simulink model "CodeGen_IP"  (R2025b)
settings: Solver=VariableStepAuto  StartTime=0.0  StopTime=10  RelTol=1e-3  EnableMultiTasking=on
undefined symbols (not defined in the file or in its folder): gray
libraries: hlsBasic x5, Sobeledge_lib x2, visionsinks x2, dspvision x1

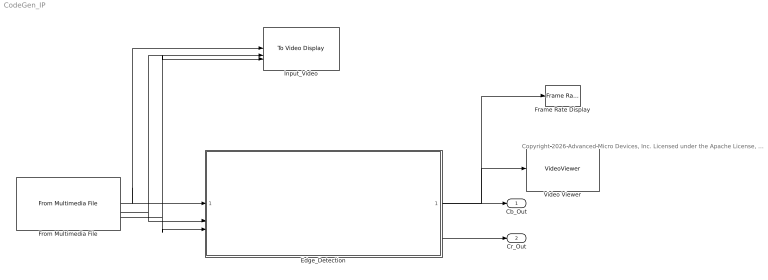
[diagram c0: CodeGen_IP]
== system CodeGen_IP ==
  note: Copyright 2026 Advanced Micro Devices, Inc. Licensed under the Apache License, Version 2.0 (the "License"); you may not use this file except in compliance with the License. You may obtain a copy of the License at http://www.apache.org/licenses/LICENSE-2.0 Unless required by applicable law or agreed to in writing, software distributed under the License is distributed on an "AS IS" BASIS, WITHOUT WARRANTIES OR CONDITIONS OF ANY KIND, either express or implied. See the License for the specific language governing permissions and limitations under the License.
  Edge_Detection : Subsystem
  Frame Rate Display : visionsinks/Frame Rate Display  UpdateRate=10
  From Multimedia File : dspvision/From Multimedia File  inputFilename=visiontraffic.avi  readRange=[1 Inf]  loop=on  numPlays=inf  outputStreams=Video only  videoDataType=uint8  audioDataType=int16  inheritSampleTime=off  userDefinedSampleTime=1/30  noAudioOutput=off  isIntensityVideo=off  fourcc=YCbCr 4:2:2  colorVideoFormat=Separate color signals  outputEOF=off  dataOrg=Column-major  audioFrameSize=1024  computeAudioFrameSize=off  outSamplingMode=Sample based
  Input_Video : visionsinks/To Video Display  windowSizeMode=Normal  openAtMdlStart=on  fullScreen=off  videoWindowX=150  videoWindowY=269  saveWindowSize=off  videoWindowWidth=581  videoWindowHeight=403  inputColorFormat=YCbCr 4:2:2  inputType=Obsolete  imagePorts=One multidimensional signal  OutputDevice=On-screen video monitor  dataOrg=Column-major  isWindowOpen=off
  Video Viewer : VideoViewer  colormapValue=gray(256)  FigPos=[755.4 772 579.6 322.8]
  Cb_Out : Outport
  Cr_Out : Outport  Port=2
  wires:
  From Multimedia File/1 -> Input_Video/1, Edge_Detection/1(Y)
  Edge_Detection/1(Y_Out) -> Video Viewer/1, Frame Rate Display/1
  From Multimedia File/2 -> Input_Video/2, Edge_Detection/2(Cb)
  From Multimedia File/3 -> Input_Video/3, Edge_Detection/3(Cr)
  Edge_Detection/3(Cr_Out) -> Cr_Out/1
  Edge_Detection/2(Cb_Out) -> Cb_Out/1

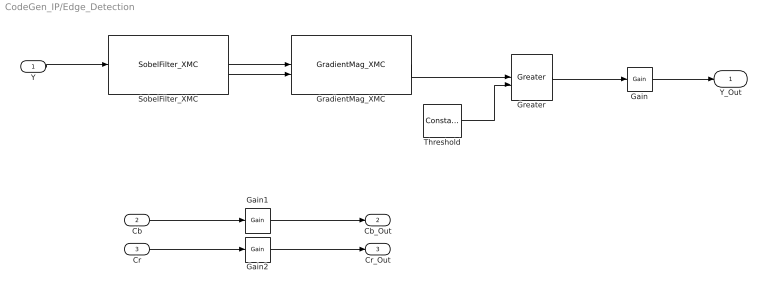
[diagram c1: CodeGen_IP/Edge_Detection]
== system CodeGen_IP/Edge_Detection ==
  Y : Inport
  Cb : Inport  Port=2
  Cr : Inport  Port=3
  Gain : hlsBasic/Gain  Gain=255  OutDataType=uint8  TypeExp=''  Signedness=Signed  WordLength=16  FractionalLength=10  RoundingMode=Truncation to minus infinity  OverflowMode=Wrap around  OutputTypeAsInput=off
  Gain1 : hlsBasic/Gain  Gain=1  OutDataType=uint8  TypeExp=''  Signedness=Signed  WordLength=16  FractionalLength=10  RoundingMode=Truncation to minus infinity  OverflowMode=Wrap around  OutputTypeAsInput=off
  Gain2 : hlsBasic/Gain  Gain=1  OutDataType=uint8  TypeExp=''  Signedness=Signed  WordLength=16  FractionalLength=10  RoundingMode=Truncation to minus infinity  OverflowMode=Wrap around  OutputTypeAsInput=off
  GradientMag_XMC : Sobeledge_lib/GradientMag_XMC  LibraryFunction=GradientMag_XMC  IncludeFiles={'GradientMag_Wrap.h'}  SourceFiles={}  IncludeDirectories={'./include'}  TemplateParams={'int ROWS'; 'int COLS'; 'int NPC'}  FunctionParamTypes={xmcDataType('void'); xmcDataType('uint16_t'); xmcDataType('uint16_t'); xmcDataType('uint16_t'); xmcDataType('int')}  FunctionParamPassbys={0.000000000000000000e+00; 0.000000000000000000e+00; 0.000000000000000000e+00; 0.000000000000000000e+00; 0.000000000000000000e+00}  FunctionParamDimensions={'1'; '[ROWS][COLS]'; '[ROWS][COLS]'; '[ROWS][COLS]'; '1'}  FunctionParamNames={'return'; 'inX'; 'inY'; 'Out'; 'NPC'}  FunctionParamDir={0.000000000000000000e+00; 1.000000000000000000e+00; 1.000000000000000000e+00; 2.000000000000000000e+00; 3.000000000000000000e+00}  FunctionParamSupportsStreaming={true; true; true; true; true}  BufferDepth={'0'}  FunctionParamValues={'0'; '0'; '0'; '0'; '0'}  ThroughputFactors={''}  NPC=1
  Greater : hlsBasic/Greater  Description=Performs multiplication
  SobelFilter_XMC : Sobeledge_lib/SobelFilter_XMC  LibraryFunction=SobelFilter_XMC  IncludeFiles={'sobelfilter_Wrap.h'}  SourceFiles={}  IncludeDirectories={'./include'}  TemplateParams={'int ROWS'; 'int COLS'; 'int NPC'}  FunctionParamTypes={xmcDataType('void'); xmcDataType('uint8_t'); xmcDataType('uint16_t'); xmcDataType('uint16_t'); xmcDataType('int')}  FunctionParamPassbys={0.000000000000000000e+00; 0.000000000000000000e+00; 0.000000000000000000e+00; 0.000000000000000000e+00; 0.000000000000000000e+00}  FunctionParamDimensions={'1'; '[ROWS][COLS]'; '[ROWS][COLS]'; '[ROWS][COLS]'; '1'}  FunctionParamNames={'return'; 'in'; 'outX'; 'outY'; 'NPC'}  FunctionParamDir={0.000000000000000000e+00; 1.000000000000000000e+00; 2.000000000000000000e+00; 2.000000000000000000e+00; 3.000000000000000000e+00}  FunctionParamSupportsStreaming={true; true; true; true; true}  BufferDepth={'0'}  FunctionParamValues={'0'; '0'; '0'; '0'; '0'}  ThroughputFactors={''}  NPC=1
  Threshold : hlsBasic/Constant  Description=Performs multiplication  Value=150  VectorParams1D=off  SampleTime=-1  OutDataType=int16  TypeExp=''  Signedness=Signed  WordLength=16  FractionalLength=0  RoundingMode=Truncation to minus infinity  OverflowMode=Wrap around
  Y_Out : Outport
  Cb_Out : Outport  Port=2
  Cr_Out : Outport  Port=3
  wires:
  Y/1 -> SobelFilter_XMC/1
  Threshold/1 -> Greater/2
  GradientMag_XMC/1 -> Greater/1
  SobelFilter_XMC/1 -> GradientMag_XMC/1
  SobelFilter_XMC/2 -> GradientMag_XMC/2
  Greater/1 -> Gain/1
  Gain/1 -> Y_Out/1
  Gain1/1 -> Cb_Out/1
  Gain2/1 -> Cr_Out/1
  Cb/1 -> Gain1/1
  Cr/1 -> Gain2/1
